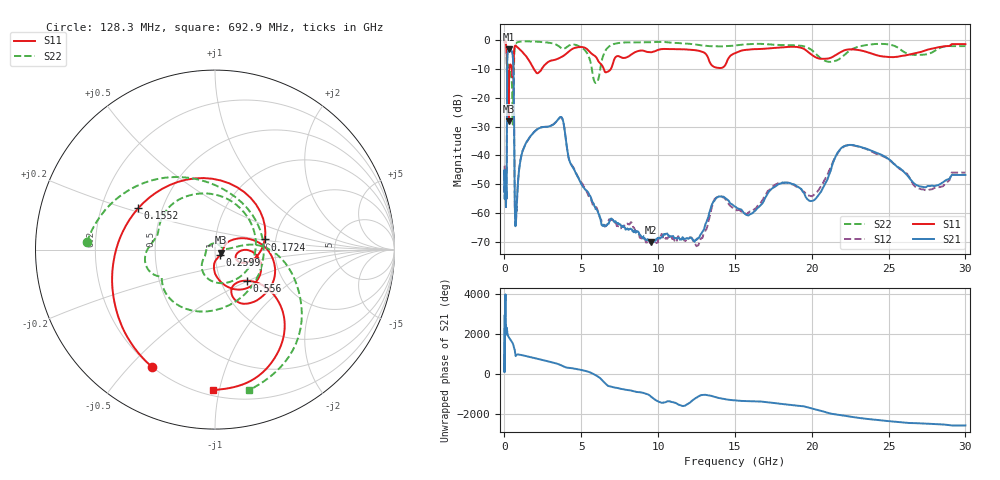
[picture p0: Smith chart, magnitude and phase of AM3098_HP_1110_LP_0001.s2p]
! Date/Time: Thu, Feb 28, 2019 8:46 AM
! Network Analyzer: Agilent Technologies E8364B Rev: A.07.50.67
! Sweep from 0.010 to 30.000 GHz, 1601 Points, Sweep Type: LOG
! Power Supply: 5.023 V, 0.002 A
# Hz S DB R 50
!freq MagS11 AngS11 MagS21 AngS21 MagS12 AngS12 MagS22 AngS22
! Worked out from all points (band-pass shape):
!   1601 points, 10 MHz to 30 GHz, reference 50 ohm
!   highest |S21| = -3.35 dB at 291.6 MHz (marker M1); lowest = -69.9 dB at 9.538 GHz (marker M2)
!   |S21| within 3 dB of the highest: 183.3 MHz to 551.8 MHz (368.5 MHz wide, 100 % of centre)
!   lowest |S11| = -28.1 dB at 263.8 MHz (marker M3), VSWR 1.08, Z = 53.6 - j1.85 ohm
!   |S11| at or under -10 dB: 170 MHz to 323.2 MHz (153.2 MHz wide, 62.1 % of centre); 1.898 GHz to 2.439 GHz (541.2 MHz wide, 25 % of centre); 6.458 GHz to 6.938 GHz (479.7 MHz wide, 7.16 % of centre)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
!   |S22| runs from -29.3 to -0.5 dB; largest |S21 - S12| = 0.011
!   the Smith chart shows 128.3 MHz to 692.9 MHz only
!   S11 on the Smith chart (normalised r, x): 128.3 MHz: 0.20, -0.58; 155.2 MHz: 0.37, +0.22; 172.4 MHz: 1.75, +0.22; 259.9 MHz: 1.05, -0.07; 556 MHz: 1.33, -0.49; 692.9 MHz: 0.24, -0.96
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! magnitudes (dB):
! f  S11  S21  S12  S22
! 10 MHz  -0.4  -45.3  -43.5  -0.5
! 38.04 MHz  -0.3  -50.7  -52.3  -0.6
! 128.3 MHz  -2.6  -54.1  -54.5  -2.9
! 144.7 MHz  -4.3  -50.8  -50.6  -5.7
! 155.2 MHz  -6.3  -34.3  -34.4  -10.4
! 172.4 MHz  -11.0  -10.8  -10.8  -8.6
! 225.9 MHz  -11.6  -3.9  -3.9  -8.2
! 259.9 MHz  -27.8  -3.4  -3.4  -9.4
! 263.8 MHz  -28.1  -3.4  -3.4  -9.5
! 291.6 MHz  -14.8  -3.3  -3.3  -9.5
! 550.5 MHz  -12.5  -6.3  -6.2  -29.0
! 556 MHz  -12.1  -6.6  -6.6  -28.0
! 605.4 MHz  -5.8  -15.6  -15.5  -11.6
! 692.9 MHz  -2.1  -62.2  -62.7  -1.9
! 2.084 GHz  -11.5  -31.2  -31.1  -0.7
! 3.704 GHz  -6.0  -26.8  -26.8  -2.9
! 5.959 GHz  -6.0  -58.5  -57.8  -15.0
! 7.926 GHz  -6.2  -65.3  -64.3  -1.0
! 9.538 GHz  -4.4  -69.9  -70.2  -0.9
! 20.1 GHz  -5.6  -55.6  -53.8  -4.1
! 22.56 GHz  -3.4  -36.3  -36.4  -3.5
! 30 GHz  -1.6  -46.7  -45.9  -2.2
